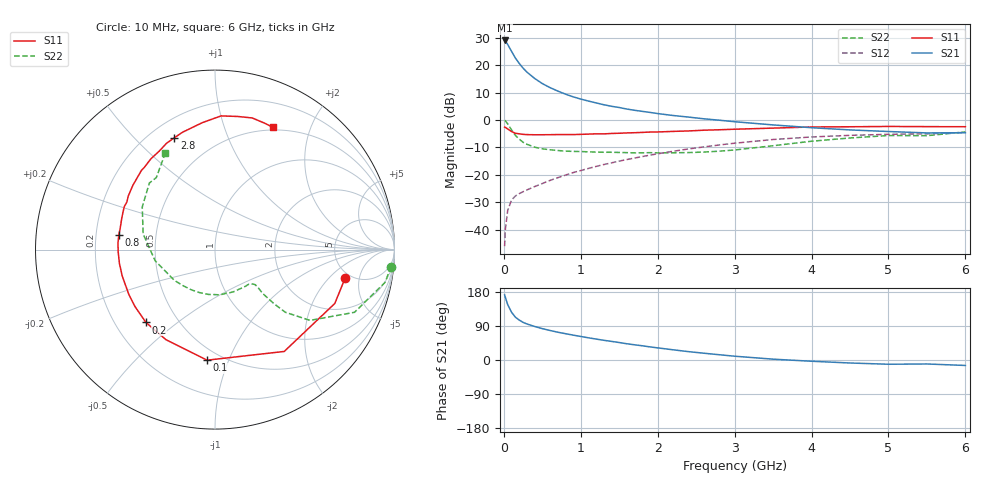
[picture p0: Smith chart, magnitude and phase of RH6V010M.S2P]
! SIEMENS Small Signal Semiconductors
! BFR106
! Si NPN RF Bipolar Junction Transistor in SOT23
! VCE = 6 V  IC = 10 mA
! Common Emitter S-Parameters:  August  1996
# GHz  S  MA  R  50
!  f  S11  S21  S12  S22
! GHz  MAG  ANG  MAG  ANG  MAG  ANG  MAG  ANG
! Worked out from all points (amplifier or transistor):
!   36 points, 10 MHz to 6 GHz, reference 50 ohm
!   highest |S21| = 29.0 dB at 10 MHz (marker M1)
!   |S21| within 3 dB of that: start of sweep to 80.74 MHz
!   unconditionally stable (mu >= 1): 486.1 MHz to 1.9 GHz; 5.335 GHz to end of sweep
!   at 250 MHz: K = 0.70, MSG = 22.5 dB, |S12| = -26.1 dB
!   at 1.4 GHz: K = 1.09, MAG = 8.5 dB, |S12| = -15.6 dB
!   at 6 GHz: K = 1.01, MAG = -0.5 dB, |S12| = -4.5 dB
!   S11 on the Smith chart (normalised r, x): 10 MHz: 4.49, -3.14; 100 MHz: 0.42, -0.84; 200 MHz: 0.33, -0.39; 800 MHz: 0.30, +0.07; 2.8 GHz: 0.30, +0.66; 6 GHz: 0.47, +1.48
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0.01  0.7426 -12.2  28.2 171.8  0.005 86.5  0.986 -5.5
0.02  0.7319 -24.2  27.58 165.2  0.0102 78.8  0.965 -10.9
0.05  0.6861 -55.8  23.84 146.3  0.0224 64.9  0.8522 -24.2
0.1  0.6176 -94.1  17.86 126.1  0.0346 53.1  0.6599 -36.7
0.15  0.5715 -118.5  13.5 113.0  0.0411 48.0  0.5249 -41.7
0.2  0.5592 -133.5  10.76 105.4  0.0454 47.4  0.448 -42.5
0.25  0.5472 -144.6  8.828 99.3  0.0493 48.0  0.3924 -42.6
0.3  0.5413 -152.4  7.471 95.1  0.053 49.8  0.3604 -42.6
0.4  0.5375 -164.1  5.726 88.5  0.061 53.0  0.3195 -41.4
0.5  0.538 -171.7  4.612 82.8  0.0694 55.5  0.2982 -41.1
0.6  0.5397 -178.7  3.897 77.9  0.079 58.3  0.2864 -42.0
0.8  0.5418 171.2  2.965 69.5  0.0987 61.1  0.2705 -45.4
0.9  0.5415 167.0  2.647 65.7  0.1097 62.3  0.2675 -47.3
1.1  0.5527 158.3  2.212 58.5  0.1308 63.2  0.2627 -53.3
1.3  0.5579 151.7  1.896 52.0  0.154 63.2  0.2578 -59.6
1.6  0.5809 142.1  1.581 42.8  0.1902 62.1  0.2538 -71.1
2.2  0.6193 125.2  1.207 26.9  0.269 57.0  0.2524 -98.4
2.8  0.6631 109.9  0.991 13.9  0.3501 48.9  0.2699 -132.5
3.5  0.7108 95.7  0.813 2.2  0.4408 37.7  0.3394 -169.5
4.5  0.7523 80.4  0.659 -7.9  0.5243 20.0  0.4699 149.6
5.5  0.7566 68.4  0.581 -10.5  0.5595 8.0  0.5175 129.2
6  0.7536 64.6  0.586 -14.4  0.5926 0.1  0.6062 117.1
